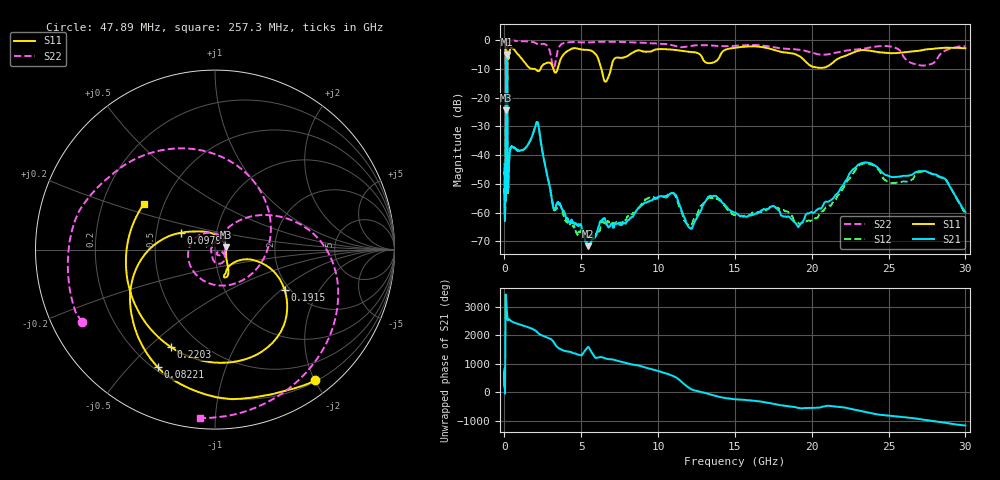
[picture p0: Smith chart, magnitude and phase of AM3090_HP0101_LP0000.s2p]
! Date/Time: Thu, Feb 28, 2019 1:58 PM
! Network Analyzer: Agilent Technologies E8364B Rev: A.07.50.67
! Sweep from 0.010 to 30.000 GHz, 1601 Points, Sweep Type: LOG
! Power Supply: 5.023 V, 0.002 A
# Hz S DB R 50
!freq MagS11 AngS11 MagS21 AngS21 MagS12 AngS12 MagS22 AngS22
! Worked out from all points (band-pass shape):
!   1601 points, 10 MHz to 30 GHz, reference 50 ohm
!   highest |S21| = -5.05 dB at 137.6 MHz (marker M1); lowest = -71.7 dB at 5.446 GHz (marker M2)
!   |S21| within 3 dB of the highest: 105.7 MHz to 175 MHz (69.24 MHz wide, 49.3 % of centre)
!   lowest |S11| = -24.4 dB at 105.1 MHz (marker M3), VSWR 1.13, Z = 56.3 + j1.36 ohm
!   |S11| at or under -10 dB: 1.957 GHz to 2.349 GHz (392.2 MHz wide, 18.2 % of centre); 3.186 GHz to 3.461 GHz (275.5 MHz wide, 8.29 % of centre); 6.308 GHz to 6.931 GHz (623.7 MHz wide, 9.42 % of centre)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
!   |S22| runs from -34.1 to -0.1 dB; largest |S21 - S12| = 0.012
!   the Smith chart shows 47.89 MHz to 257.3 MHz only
!   S11 on the Smith chart (normalised r, x): 47.89 MHz: 0.22, -2.01; 82.21 MHz: 0.22, -0.61; 97.94 MHz: 0.67, +0.13; 191.5 MHz: 1.88, -1.05; 220.3 MHz: 0.35, -0.59; 257.3 MHz: 0.39, +0.25
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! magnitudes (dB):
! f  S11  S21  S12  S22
! 10 MHz  -0.3  -43.1  -44.7  -0.4
! 38.04 MHz  -0.5  -59.8  -60.2  -1.2
! 47.89 MHz  -0.8  -52.2  -49.2  -1.5
! 82.21 MHz  -2.7  -46.1  -46.2  -5.9
! 97.94 MHz  -13.4  -14.5  -14.5  -14.9
! 105.1 MHz  -24.4  -8.3  -8.4  -18.3
! 137.6 MHz  -16.5  -5.1  -5.0  -32.3
! 144.7 MHz  -16.9  -5.1  -5.1  -24.1
! 170.7 MHz  -16.2  -7.1  -7.0  -33.1
! 191.5 MHz  -7.0  -22.3  -22.2  -8.5
! 220.3 MHz  -4.5  -51.2  -53.3  -1.3
! 257.3 MHz  -6.5  -49.4  -49.8  -0.5
! 550.5 MHz  -3.0  -37.2  -37.4  -0.2
! 2.084 GHz  -10.4  -28.8  -28.7  -1.2
! 3.236 GHz  -10.8  -59.0  -58.9  -9.4
! 5.446 GHz  -3.4  -71.7  -68.4  -0.8
! 6.619 GHz  -14.4  -63.9  -64.1  -0.6
! 7.926 GHz  -5.8  -63.2  -62.5  -0.7
! 10.76 GHz  -3.3  -53.6  -53.4  -1.6
! 19.61 GHz  -7.5  -60.7  -63.2  -3.8
! 23.48 GHz  -3.5  -42.6  -42.9  -2.9
! 30 GHz  -2.8  -59.8  -60.5  -2.2
